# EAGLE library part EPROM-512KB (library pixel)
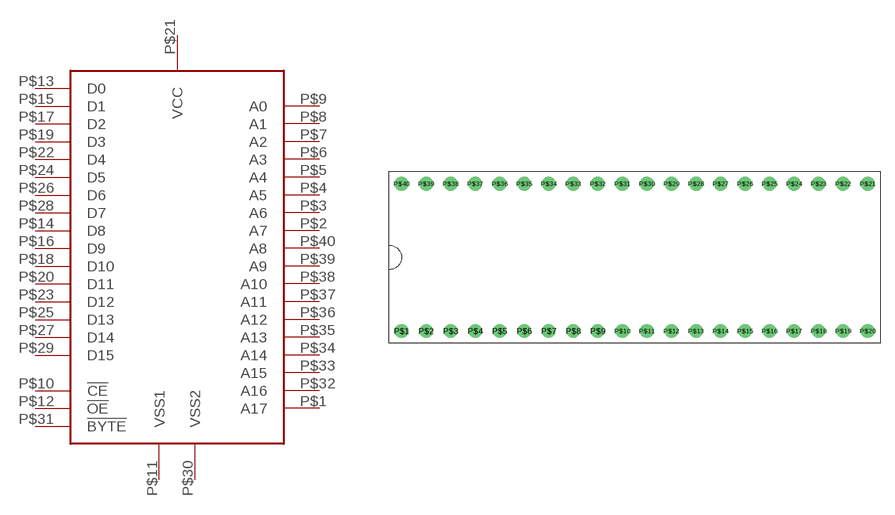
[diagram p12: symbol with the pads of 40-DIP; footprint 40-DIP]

Designator prefix -

## EPROM-512KB  [40-DIP]
P$1  A17
P$2  A7
P$3  A6
P$4  A5
P$5  A4
P$6  A3
P$7  A2
P$8  A1
P$9  A0
P$10  !CE
P$11  VSS1
P$12  !OE
P$13  D0
P$14  D8
P$15  D1
P$16  D9
P$17  D2
P$18  D10
P$19  D3
P$20  D11
P$21  VCC
P$22  D4
P$23  D12
P$24  D5
P$25  D13
P$26  D6
P$27  D14
P$28  D7
P$29  D15
P$30  VSS2
P$31  !BYTE
P$32  A16
P$33  A15
P$34  A14
P$35  A13
P$36  A12
P$37  A11
P$38  A10
P$39  A9
P$40  A8

## Footprint 40-DIP (pad centres in mm)
drill 0.9: P$1 -24.13,-7.62; P$2 -21.59,-7.62; P$3 -19.05,-7.62; P$4 -16.51,-7.62; P$5 -13.97,-7.62; P$6 -11.43,-7.62; P$7 -8.89,-7.62; P$8 -6.35,-7.62; P$9 -3.81,-7.62; P$10 -1.27,-7.62; P$11 1.27,-7.62; P$12 3.81,-7.62; P$13 6.35,-7.62; P$14 8.89,-7.62; P$15 11.43,-7.62; P$16 13.97,-7.62; P$17 16.51,-7.62; P$18 19.05,-7.62; P$19 21.59,-7.62; P$20 24.13,-7.62; P$21 24.13,7.62; P$22 21.59,7.62; P$23 19.05,7.62; P$24 16.51,7.62; P$25 13.97,7.62; P$26 11.43,7.62; P$27 8.89,7.62; P$28 6.35,7.62; P$29 3.81,7.62; P$30 1.27,7.62; P$31 -1.27,7.62; P$32 -3.81,7.62; P$33 -6.35,7.62; P$34 -8.89,7.62; P$35 -11.43,7.62; P$36 -13.97,7.62; P$37 -16.51,7.62; P$38 -19.05,7.62; P$39 -21.59,7.62; P$40 -24.13,7.62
